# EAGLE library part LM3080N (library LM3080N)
IC OP TRANSCONDUCTIVE AMP 8DIP Source: Datasheet
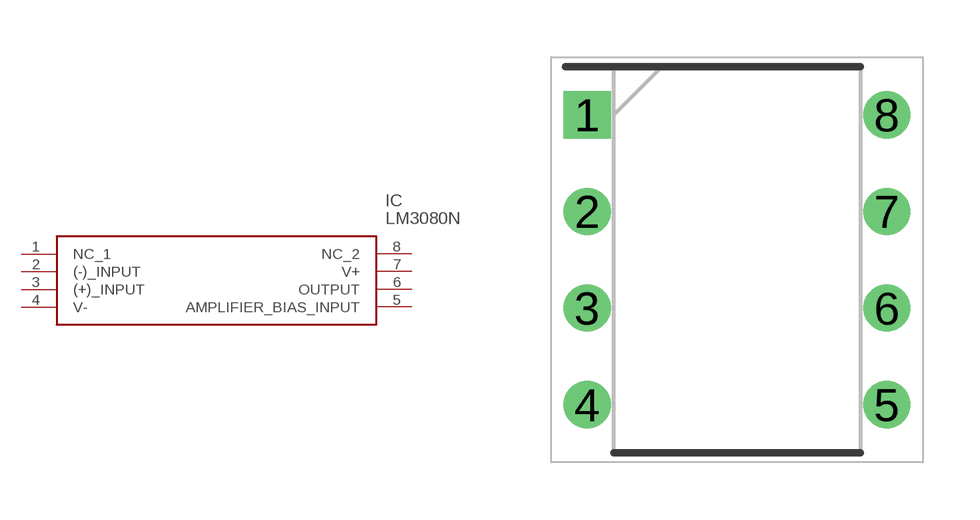
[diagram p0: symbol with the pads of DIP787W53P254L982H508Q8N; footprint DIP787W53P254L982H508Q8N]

Designator prefix IC

## LM3080N (Description: IC OP TRANSCONDUCTIVE AMP 8DIP; Height: 5.08mm; Manufacturer_Name: Texas Instruments; Manufacturer_Part_Number: LM3080N; Mouser_Part_Number: N/A; Mouser_Price-Stock: https://www.mouser.com/Search/Refine.aspx?Keyword=N%2FA)  [DIP787W53P254L982H508Q8N]
1  NC_1
2  (-)_INPUT
3  (+)_INPUT
4  V-
5  AMPLIFIER_BIAS_INPUT
6  OUTPUT
7  V+
8  NC_2

## Footprint DIP787W53P254L982H508Q8N (pad centres in mm)
Molded Dual-In-Line Package (N) Order Number LM6265N or LM6365N NS Package Number N08E
drill 0.733 pad 1.133 square: 1 -3.937,3.81
drill 0.733 pad 1.133: 2 -3.937,1.27; 3 -3.937,-1.27; 4 -3.937,-3.81; 5 3.937,-3.81; 6 3.937,-1.27; 7 3.937,1.27; 8 3.937,3.81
